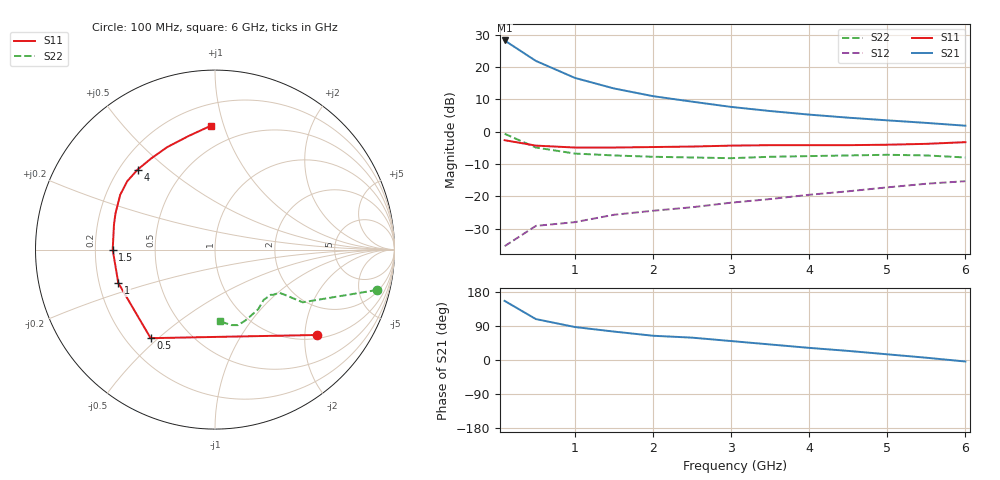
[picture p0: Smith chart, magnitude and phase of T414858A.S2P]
!AT-41485
!S-PARAMETERS at Vce=8V  Ic=10mA.  LAST UPDATED 07-21-92
# ghz s ma r 50
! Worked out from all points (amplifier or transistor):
!   13 points, 100 MHz to 6 GHz, reference 50 ohm
!   highest |S21| = 28.2 dB at 100 MHz (marker M1)
!   |S21| within 3 dB of that: start of sweep to 289.8 MHz
!   unconditionally stable (mu >= 1): 1.372 GHz to 5.212 GHz
!   at 1 GHz: K = 0.92, MSG = 22.3 dB, |S12| = -28.0 dB
!   at 3 GHz: K = 1.24, MAG = 11.9 dB, |S12| = -21.9 dB
!   at 6 GHz: K = 0.92, MSG = 8.6 dB, |S12| = -15.3 dB
!   lowest NFmin = 1.30 dB at 100 MHz
!   S11 on the Smith chart (normalised r, x): 100 MHz: 1.09, -2.30; 500 MHz: 0.30, -0.47; 1 GHz: 0.28, -0.15; 1.5 GHz: 0.27, -0.00; 4 GHz: 0.27, +0.40; 6 GHz: 0.34, +0.90
0.1  0.74 -40.0  25.8 156.0  0.017 81.0  0.93 -14.0
0.5  0.61 -126.0  12.46 108.0  0.035 44.0  0.57 -31.0
1  0.57 -161.0  6.8 87.0  0.04 38.0  0.46 -33.0
1.5  0.57 -180.0  4.67 75.0  0.052 47.0  0.43 -34.0
2  0.58 166.0  3.55 64.0  0.06 54.0  0.41 -38.0
2.5  0.59 160.0  2.92 59.0  0.068 58.0  0.4 -39.0
3  0.61 150.0  2.42 50.0  0.08 63.0  0.39 -46.0
3.5  0.62 142.0  2.09 41.0  0.091 61.0  0.41 -54.0
4  0.62 134.0  1.84 32.0  0.106 59.0  0.42 -62.0
4.5  0.62 125.0  1.65 24.0  0.12 57.0  0.43 -67.0
5  0.63 115.0  1.5 15.0  0.138 54.0  0.44 -73.0
5.5  0.65 103.0  1.37 6.0  0.157 49.0  0.43 -78.0
6  0.69 92.0  1.24 -4.0  0.172 46.0  0.4 -86.0
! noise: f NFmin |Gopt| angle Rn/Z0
0.1  1.3  0.12  5  0.17
0.5  1.3  0.1  25  0.17
1  1.4  0.06  50  0.16
2  1.7  0.25  172  0.16
4  3  0.48  -131  0.24
